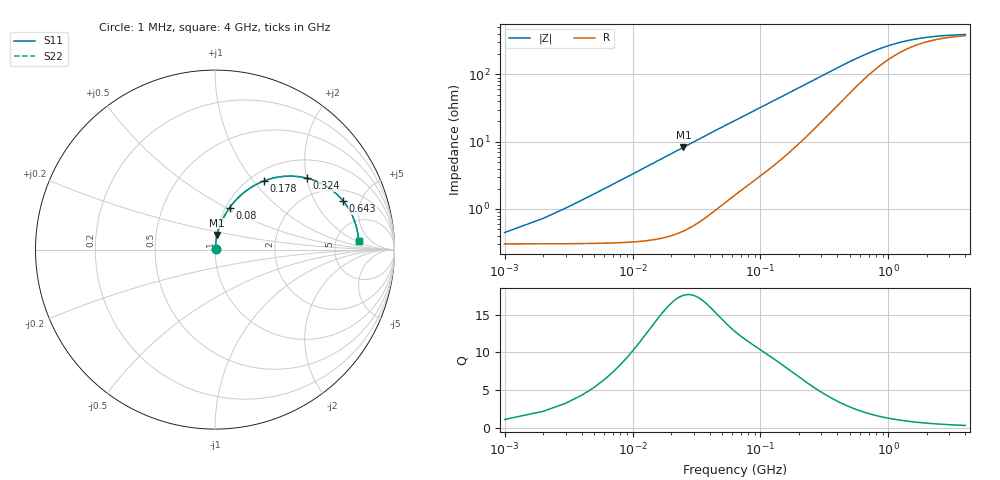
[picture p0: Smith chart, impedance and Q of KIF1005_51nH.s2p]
!version-2
!date-12.2020
!Series
# MHz S RI R 50
!Freq ReS11 ImS11 ReS21 ImS21 ReS12 ImS12 ReS22 ImS22
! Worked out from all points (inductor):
!   4000 points, 1 MHz to 4 GHz, reference 50 ohm
!   read as one part in series: L = 52.6 nH near 21 MHz
!   highest Q = 13.7 at 25 MHz (marker M1), where L = 52.6 nH
!   S11 on the Smith chart (normalised r, x): 1 MHz: 1.01, +0.01; 80 MHz: 1.05, +0.52; 178 MHz: 1.15, +1.13; 324 MHz: 1.46, +2.00; 643 MHz: 2.69, +3.50; 4 GHz: 8.56, +2.20
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1  0.00302 0.00327  0.997 -0.00327  0.997 -0.00327  0.00302 0.00327
11  0.00456 0.0359  0.9954 -0.0359  0.9954 -0.0359  0.00456 0.0359
22  0.00941 0.0716  0.9906 -0.0716  0.9906 -0.0716  0.00941 0.0716
25  0.0114 0.0813  0.9886 -0.0813  0.9886 -0.0813  0.0114 0.0813
34  0.0188 0.1095  0.9812 -0.1095  0.9812 -0.1095  0.0188 0.1095
46  0.0318 0.1452  0.9682 -0.1452  0.9682 -0.1452  0.0318 0.1452
61  0.0517 0.1862  0.9483 -0.1862  0.9483 -0.1862  0.0517 0.1862
80  0.081 0.2327  0.919 -0.2327  0.919 -0.2327  0.081 0.2327
100  0.116 0.2755  0.884 -0.2755  0.884 -0.2755  0.116 0.2755
123  0.1598 0.3167  0.8402 -0.3167  0.8402 -0.3167  0.1598 0.3167
178  0.2708 0.3817  0.7292 -0.3817  0.7292 -0.3817  0.2708 0.3817
243  0.3925 0.4087  0.6075 -0.4087  0.6075 -0.4087  0.3925 0.4087
324  0.5113 0.3982  0.4887 -0.3982  0.4887 -0.3982  0.5113 0.3982
463  0.6369 0.342  0.3631 -0.342  0.3631 -0.342  0.6369 0.342
643  0.7145 0.2706  0.2855 -0.2706  0.2855 -0.2706  0.7145 0.2706
668  0.7211 0.2622  0.2789 -0.2622  0.2789 -0.2622  0.7211 0.2622
963  0.7653 0.1886  0.2347 -0.1886  0.2347 -0.1886  0.7653 0.1886
1334  0.7844 0.1373  0.2156 -0.1373  0.2156 -0.1373  0.7844 0.1373
2001  0.7953 0.0917  0.2047 -0.0917  0.2047 -0.0917  0.7953 0.0917
2667  0.7988 0.0687  0.2012 -0.0687  0.2012 -0.0687  0.7988 0.0687
3334  0.8005 0.055  0.1995 -0.055  0.1995 -0.055  0.8005 0.055
4000  0.8013 0.0458  0.1987 -0.0458  0.1987 -0.0458  0.8013 0.0458
